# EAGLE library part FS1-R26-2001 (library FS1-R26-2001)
I/O Connectors MINI SAS 30 GOLD., Source: Datasheet
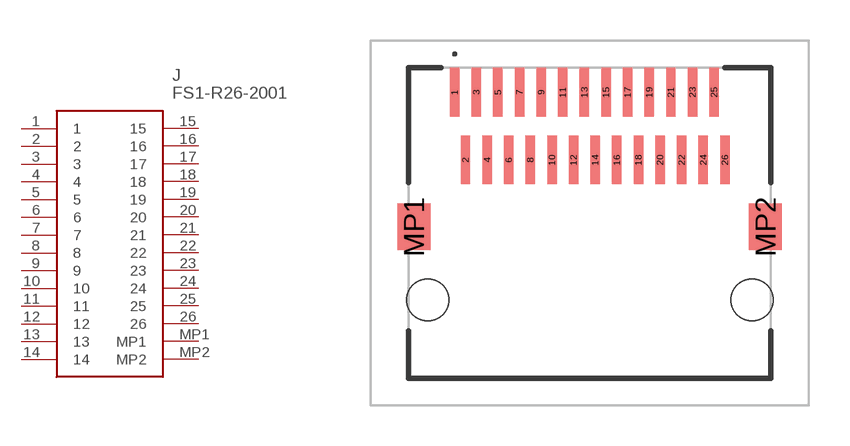
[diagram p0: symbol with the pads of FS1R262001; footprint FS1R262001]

Designator prefix J

## FS1-R26-2001 (Description: I/O Connectors MINI SAS 30 GOLD.,; Height: 5.48mm; Manufacturer_Name: Amphenol; Manufacturer_Part_Number: FS1-R26-2001; Mouser_Part_Number: 523-FS1-R26-2001; Mouser_Price-Stock: https://www.mouser.com/Search/Refine.aspx?Keyword=523-FS1-R26-2001)  [FS1R262001]
1  1
2  2
3  3
4  4
5  5
6  6
7  7
8  8
9  9
10  10
11  11
12  12
13  13
14  14
15  15
16  16
17  17
18  18
19  19
20  20
21  21
22  22
23  23
24  24
25  25
26  26
MP1  MP1
MP2  MP2

## Footprint FS1R262001 (pad centres in mm)
FS1-R26-2001-2
smd 0.35 x 1.8: 1 -4.995,4.84; 2 -4.595,2.33; 3 -4.195,4.84; 4 -3.795,2.33; 5 -3.395,4.84; 6 -2.995,2.33; 7 -2.595,4.84; 8 -2.195,2.33; 9 -1.795,4.84; 10 -1.395,2.33; 11 -0.995,4.84; 12 -0.595,2.33; 13 -0.195,4.84; 14 0.205,2.33; 15 0.605,4.84; 16 1.005,2.33; 17 1.405,4.84; 18 1.805,2.33; 19 2.205,4.84; 20 2.605,2.33; 21 3.005,4.84; 22 3.405,2.33; 23 3.805,4.84; 24 4.205,2.33; 25 4.605,4.84; 26 5.005,2.33
smd 1.22 x 1.72: MP1 -6.505,-0.15; MP2 6.505,-0.15
hole 1.55 at -5.995,-2.85
hole 1.55 at 6.005,-2.85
